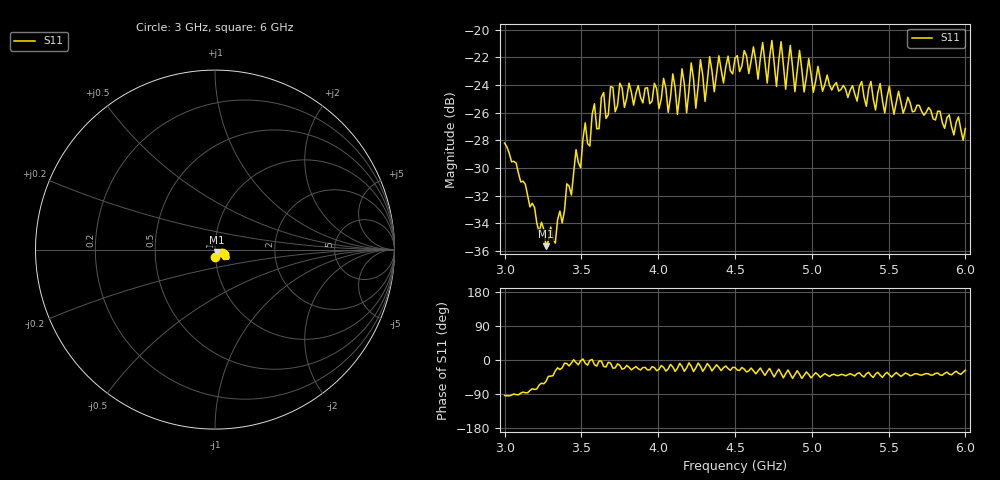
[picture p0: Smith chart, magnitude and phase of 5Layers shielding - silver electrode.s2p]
!  03/07/2025  16:14:39
! Ref Plane: 0.000 mm
# MHZ S MA R  50
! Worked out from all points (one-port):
!   201 points, 3 GHz to 6 GHz, reference 50 ohm
!   lowest |S11| = -35.6 dB at 3.27 GHz (marker M1), VSWR 1.03, Z = 50.9 - j1.39 ohm
!   |S11| at or under -10 dB: start of sweep to end of sweep
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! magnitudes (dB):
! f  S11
! 3 GHz  -28.2
! 3.27 GHz  -35.6
! 3.375 GHz  -34.0
! 3.525 GHz  -26.7
! 3.555 GHz  -28.4
! 3.585 GHz  -25.4
! 3.615 GHz  -27.1
! 3.75 GHz  -23.9
! 4.005 GHz  -25.7
! 4.035 GHz  -23.5
! 4.065 GHz  -26.0
! 4.095 GHz  -23.2
! 4.125 GHz  -26.1
! 4.155 GHz  -22.8
! 4.185 GHz  -26.0
! 4.215 GHz  -22.4
! 4.245 GHz  -25.7
! 4.275 GHz  -22.2
! 4.305 GHz  -25.2
! 4.335 GHz  -22.0
! 4.365 GHz  -24.5
! 4.395 GHz  -21.9
! 4.425 GHz  -23.9
! 4.5 GHz  -22.1
! 4.875 GHz  -22.7
! 5.25 GHz  -24.4
! 5.625 GHz  -24.9
! 6 GHz  -27.1
